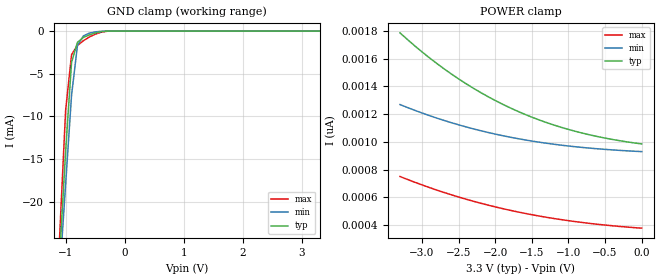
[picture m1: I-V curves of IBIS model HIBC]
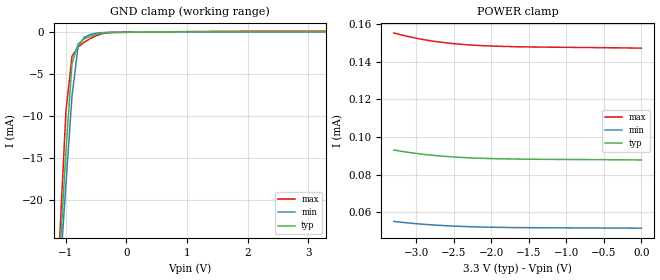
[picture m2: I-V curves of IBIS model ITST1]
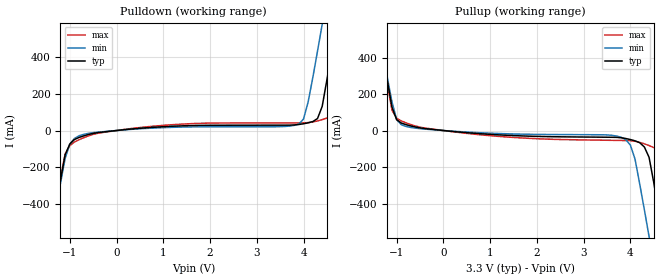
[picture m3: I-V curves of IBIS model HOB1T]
[IBIS Ver]   2.1
[Comment Char]   |_char
[File name]   a5-pfbga.ibs
[File Rev]   1.0
[Date]   2003/06/02
[Source]
[Notes]
[Disclaimer]
This information is for modelingpurposes only, and is not guaranteed.
[Copyright]
Copyright 2002, SEIKO EPSON Corp.
[Component]   S1D13a05
[Manufacturer]   SEIKO EPSON Corp.
| PFBGA-121
| PFBGA-121
[Package]
R_pkg   123.94m   113.54m   202.71m
L_pkg   0.577n   0.256n   2.951n
C_pkg   0.548p   0.443p   1.442p
[Pin] signal_name   model_name
2B   VSS   GND
3C   AB3   HIBC
2C   COREVDD   POWER
3D   AB2   HIBC
2D   AB1   HIBC
6D   AB17   HIBC
1D   AB0   HIBT
4E   CS#   HIBC
3E   M/R#   HIBT
2E   BS#   HIBT
1E   RD#   HIBT
5E   WE0#   HIBT
6E   AB13   HIBC
2F   VSS   GND
1F   RESET#   HIBT
3F   RD/WR#   HIBT
4F   WE1#   HIBT
5F   CLKI   HIBC
1G   WAIT#   HBT2T
2G   DB15   HBT2T
3G   DB14   HBT2T
4G   IOVDD   POWER
1H   DB12   HBT2T
2H   DB11   HBT2T
3H   DB10   HBT2T
4H   DB13   HBT2T
2J   DB9   HBT2T
3J   DB6   HBT2T
2K   VSS   GND
2L   IOVDD   POWER
3K   DB8   HBT2T
3L   DB7   HBT2T
4J   DB5   HBT2T
4K   DB4   HBT2T
5J   DB2   HBT2T
4L   DB3   HBT2T
5K   DB1   HBT2T
5L   DB0   HBT2T
5G   VSS   GND
1K   GPO0   HOB1T
1J   GPO1   HOB1T
5H   GPO2   HOB1T
6H   IOVDD   POWER
6J   GPO3   HOB1T
6L   GPIO7   US_P
6K   GPIO6   US_M
6G   GPIO5   HBA1T
6F   GPO4   HOB1T
7K   GPIO2   HBA1T
7L   GPIO3   HBA1T
7J   GPIO1   HBA1T
7H   GPIO4   HBA1T
7G   FPDAT5   HBT2T
8L   GPIO0   HBA1T
8K   IRQ   HOB1T
8J   USBCLK   HIBC
9L   IOVDD   POWER
9K   DRDY   HOB1T
10K   VSS   GND
10L   COREVDD   POWER
11K   GPO6   HOB1T
11J   GPO7   HOB1T
10   JCOREVDD   POWER
9J   FPFRAME   HBT2T
8H   GPO5   HOB1T
9H   FPLINE   HBT2T
10H   FPSHIFT   HBT2T
11H   FPDAT0   HBT2T
8G   FPDAT1   HBT2T
9G   FPDAT2   HBT2T
10G   FPDAT3   HBT2T
11G   FPDAT4   HBT2T
8F   FPDAT6   HBT2T
9F   VSS   GND
10F   FPDAT7   HBT2T
11F   IOVDD   POWER
7F   FPDAT8   HBT2T
9E   FPDAT12   HBT2T
10E   FPDAT11   HBT2T
11E   FPDAT10   HBT2T
8E   FPDAT9   HBT2T
7E   TESTEN   ITST1
10D   FPDAT15   HBT2T
11D   FPDAT14   HBT2T
9D   FPDAT16   HBT2T
9C   CNF6   HIBC
10C   FPDAT17   HBT2T
11C   GPO8   HOB1T
10B   VSS   GND
11B   GPO9   HOB1T
10A   IOVDD   POWER
9B   CLKI2   HIBC
9A   PWMOUT   HOB1T
8D   FPDAT13   HBT2T
8C   CNF5   HIBC
8B   CNF4   HIBC
7D   CNF3   HIBC
7C   CNF2   HIBC
7B   CNF1   HIBC
7A   CNF0   HIBC
4B   GPO10   HOB1T
1C   USBOSCO   OSCBC2
1B   USBOSCI   LLIN
6C   AB16   HIBC
6A   AB15   HIBC
6B   AB14   HIBC
5D   AB12   HIBC
5C   AB9   HIBC
5A   AB11   HIBC
5B   AB10   HIBC
4C   AB6   HIBC
4A   AB7   HIBC
4D   AB8   HIBC
3B   AB5   HIBC
3A   AB4   HIBC
2A   COREVDD   POWER
| Models and submodels in the file (10): HIBC (Input), HIBT (Input), ITST1 (Input), HOB1T (Output), HBT2T (I/O), HBA1T (I/O), OSCBC2 (Output), US_M (I/O), US_P (I/O), LLIN (Input)
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[Model]   HIBC
Model_type Input
Vinh=2.0
Vinl=0.8
C_comp   5p   4p   6p
[Temperature Range] 50   100   0
[Voltage Range]   3.3   3.0   3.6
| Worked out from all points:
|   GND clamp passes 1 mA (typ) near -0.74 V on its own axis
[GND Clamp]
-3.3V     -310.4mA   -271.5mA   -364.3mA
-1.1V     -26.25mA   -28.4mA    -23.85mA
-1V       -14.07mA   -17.95mA   -9.285mA
-900mV    -3.667mA   -7.529mA   -2.767mA
-800mV    -1.326mA   -1.694mA   -1.687mA
-700mV    -753.9uA   -566.6uA   -1.131mA
-600mV    -445.2uA   -244.2uA   -699.4uA
-500mV    -223.9uA   -92.7uA    -365.2uA
-300mV    -11.88uA   -2.451uA   -21.75uA
3.3V      985.3pA    938.7pA    367.6pA
[POWER Clamp]
-3.3V     1.786nA    1.269nA    750.1pA
-3V       1.649nA    1.208nA    689.7pA
-2.8V     1.566nA    1.172nA    652.8pA
-2.6V     1.49nA     1.139nA    618.5pA
-2.4V     1.42nA     1.108nA    586.9pA
-2.2V     1.356nA    1.081nA    557.8pA
-2V       1.298nA    1.056nA    531.1pA
-1.8V     1.246nA    1.034nA    506.9pA
-1.4V     1.158nA    997.9pA    465.1pA
-1V       1.09nA     970.3pA    431.7pA
-500mV    1.027nA    946pA      400.1pA
0V        985.3pA    929.8pA    377.7pA
[Model]   ITST1
Model_type Input
Vinh=2.0
Vinl=0.8
C_comp   5p   4p   6p
[Temperature Range] 50   100   0
[Voltage Range]   3.3   3.0   3.6
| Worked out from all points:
|   GND clamp passes 1 mA (typ) near -0.73 V on its own axis
[GND Clamp]
-3.3V     -318.7mA   -279.8mA   -372.6mA
-1.1V     -26.51mA   -28.74mA   -24.06mA
-1V       -14.19mA   -18.1mA    -9.398mA
-900mV    -3.737mA   -7.598mA   -2.856mA
-800mV    -1.383mA   -1.738mA   -1.765mA
-700mV    -801.8uA   -601.7uA   -1.199mA
-600mV    -485.9uA   -273.4uA   -757.4uA
-500mV    -257.5uA   -116.6uA   -413.2uA
-300mV    -31.62uA   -16.38uA   -50.27uA
3.3V      87.75uA    51.52uA    146.9uA
[POWER Clamp]
-3.3V     93.04uA    55.05uA    155.3uA
-3.2V     92.36uA    54.61uA    154.3uA
-3.1V     91.75uA    54.21uA    153.3uA
-3V       91.21uA    53.84uA    152.5uA
-2.8V     90.31uA    53.24uA    151.1uA
-2.7V     89.93uA    52.98uA    150.5uA
-2.5V     89.34uA    52.57uA    149.6uA
-2.4V     89.1uA     52.41uA    149.3uA
-2.2V     88.73uA    52.15uA    148.7uA
-1.9V     88.38uA    51.89uA    148.2uA
-1.6V     88.19uA    51.75uA    147.9uA
0V        87.75uA    51.47uA    147.2uA
[Model]   HOB1T
Model_type Output
Polarity Non-Inverting
C_comp   5p   4p   6p
[Temperature Range] 50   100   0
[Voltage Range]   3.3   3.0   3.6
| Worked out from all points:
|   slope of the pulldown table from 0 to 0.495 V, typ, clamps not added: 40.5 ohm
|   slope of the pullup table from 0 to 0.495 V, typ, clamps not added: 42.6 ohm
[Pullup]
-3.3V     3.687A     3.389A     4.049A
-1.4V     592.9mA    581.8mA    608.6mA
-1.1V     128mA      156.1mA    110.8mA
-900mV    41.08mA    31.54mA    52.69mA
900mV     -19.27mA   -13.49mA   -25.91mA
3.6V      -36.94mA   -26.11mA   -53.67mA
3.9V      -43.64mA   -50.13mA   -54.8mA
4.1V      -56.52mA   -157mA     -58.91mA
4.4V      -146.8mA   -581mA     -82.35mA
4.7V      -601.7mA   -1.02A     -154.8mA
5V        -1.087A    -1.46A     -634.1mA
6.6V      -3.692A    -3.821A    -3.546A
[Pulldown]
-3.3V     -3.684A    -3.376A    -4.079A
-1.4V     -591.9mA   -578.3mA   -616.1mA
-1.1V     -133.3mA   -152.9mA   -128.3mA
-800mV    -37.62mA   -28.47mA   -50.17mA
3.9V      33.09mA    35.69mA    41.78mA
4.1V      42.11mA    157.5mA    43.49mA
4.3V      65.66mA    435mA      52.54mA
4.4V      132.3mA    581.6mA    59.65mA
4.5V      276.6mA    728.4mA    68.34mA
4.7V      595.1mA    1.022A     121.9mA
5V        1.082A     1.464A     615.3mA
6.6V      3.687A     3.828A     3.513A
[Ramp]
R_load=50
dV/dt_r   9.122E-1/3.137E-10   6.298E-1/3.911E-10   1.191E+0/2.564E-10
dV/dt_f   8.547E-1/4.090E-10   6.141E-1/4.860E-10   1.153E+0/3.602E-10
